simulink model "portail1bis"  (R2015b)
settings: Solver=FixedStepDiscrete  StartTime=0.0  StopTime=inf  RelTol=1e-3
libraries: realtime_pacer_lib x1

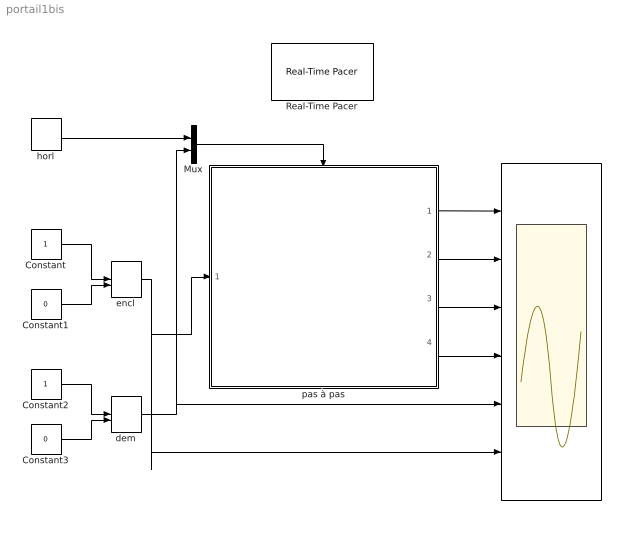
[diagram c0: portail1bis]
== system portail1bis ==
  " " : Scope  NumInputPorts=6
  Constant : Constant
  Constant1 : Constant  Value=0
  Constant2 : Constant
  Constant3 : Constant  Value=0
  Mux : Mux  Inputs=2
  Real-Time Pacer : realtime_pacer_lib/Real-Time Pacer  simTimePerRealTime=1
  dem : ManualSwitch  CurrentSetting=0
  encl : ManualSwitch
  horl : DiscretePulseGenerator  PulseType=Time based  Period=0.1  PulseWidth=5
  pas à pas : Stateflow chart  TreatAsAtomicUnit=on
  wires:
  Constant/1 -> encl/1
  Constant1/1 -> encl/2
  Constant2/1 -> dem/1
  Constant3/1 -> dem/2
  pas à pas/1(CGV) -> " "/1
  pas à pas/2(SGV) -> " "/2
  pas à pas/4(SPV) -> " "/4
  encl/1 -> pas à pas/1(encl), " "/6
  dem/1 -> Mux/2, " "/5
  pas à pas/3(CPV) -> " "/3
  horl/1 -> Mux/1
  Mux/1 -> pas à pas/Trigger

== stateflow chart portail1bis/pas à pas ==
  state portail_arrete
    du:CGV=0;
    SGV=0;
    CPV=0;
    SPV=0;
  state portail_marche_pas
    state ouverture
      du:CGV=150;
      SGV=0;
      CPV=150;
      SPV=0;
    state arret
      du:CGV=0;
      SGV=0;
      CPV=0;
      SPV=0;
    state fermeture
      du:CGV=150;
      SGV=1;
      CPV=150;
      SPV=1;
    state arret1
      du:CGV=0;
      SGV=0;
      CPV=0;
      SPV=0;
    (default) -> arret
    fermeture -> arret : dem
    arret -> ouverture : dem
    ouverture -> arret1 : dem
    arret1 -> fermeture : dem
  (default) -> portail_arrete
  portail_marche_pas -> portail_arrete : [!encl]
  portail_arrete -> portail_marche_pas : [encl]
  data: CGV output; SGV output; CPV output; SPV output; encl input
  events: input RISING_EDGE_EVENT; input RISING_EDGE_EVENT
